FUNCTION_BLOCK FB_DO_IED_LD1_LPHD1_PhyNam EXTENDS FB_AcsiCommonDataClass
VAR_INPUT
	vendor: FB_AcsiDATypeVisString255 := (fc:=ACSI_FC_DC, sValue:='Beckhoff Automation', bLinkResult:=THIS^.AddDataToContainer(ipData:=vendor));
	hwRev: FB_AcsiDATypeVisString255 := (fc:=ACSI_FC_DC, sValue:='1.0', bLinkResult:=THIS^.AddDataToContainer(ipData:=hwRev));
	swRev: FB_AcsiDATypeVisString255 := (fc:=ACSI_FC_DC, sValue:='1.0', bLinkResult:=THIS^.AddDataToContainer(ipData:=swRev));
	serNum: FB_AcsiDATypeVisString255 := (fc:=ACSI_FC_DC, sValue:='00000001', bLinkResult:=THIS^.AddDataToContainer(ipData:=serNum));
	model: FB_AcsiDATypeVisString255 := (fc:=ACSI_FC_DC, sValue:='Demo LPHD', bLinkResult:=THIS^.AddDataToContainer(ipData:=model));
	location: FB_AcsiDATypeVisString255 := (fc:=ACSI_FC_DC, sValue:='Verl', bLinkResult:=THIS^.AddDataToContainer(ipData:=location));
END_VAR
VAR
END_VAR

END_FUNCTION_BLOCK
